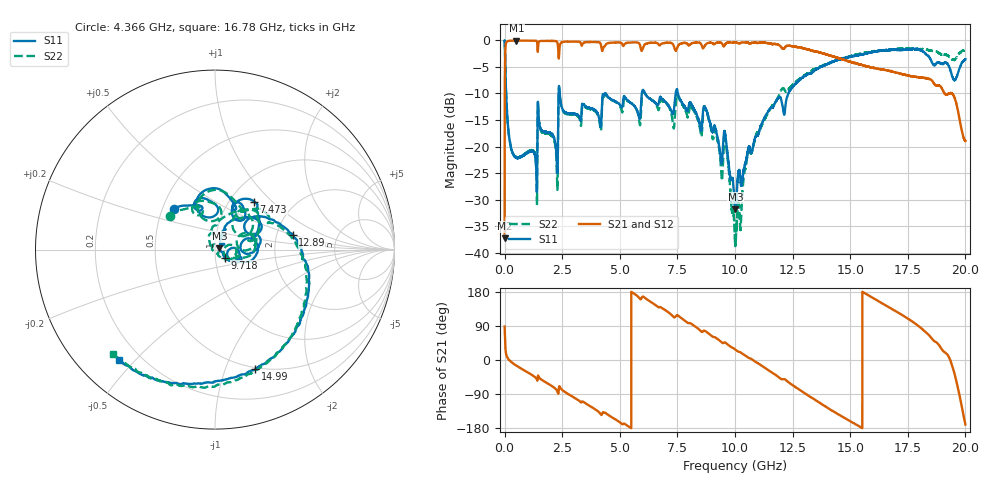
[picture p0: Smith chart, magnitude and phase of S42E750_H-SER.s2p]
!{S42E750}
!Johanson Technology Inc.
!www.johansontechnology.com
!Test Board Conditions:
!Substrate Type  RO4350B
!Substrate Thickness  50 mil
!Substrate Dk  3.66
!TL Type: GCPW
!TL Trace Width  60 mil
!TL Gap  10 mil
!Electrode orientation  Horizontal
!DUT TOPOLOGY	SERIES
!Mounting Pad LxW  14x55 mil
! Created Wed Nov 25 22:25:57 2020
# khz S ma R 50
! 2 Port Network Data from SP1.SP block
! freq  magS11  angS11  magS21  angS21  magS12  angS12  magS22  angS22
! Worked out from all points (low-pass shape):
!   20001 points, 300 kHz to 20 GHz, reference 50 ohm
!   highest |S21| = -0.04 dB at 511.3 MHz (marker M1); lowest = -37.3 dB at 300 kHz (marker M2)
!   |S21| within 3 dB of the highest: 21.74 MHz to 2.342 GHz (2.32 GHz wide, 196 % of centre); 2.36 GHz to 14.25 GHz (11.89 GHz wide, 143 % of centre)
!   lowest |S11| = -31.8 dB at 10.02 GHz (marker M3), VSWR 1.05, Z = 52.5 + j0.76 ohm
!   |S11| at or under -10 dB: 65.96 MHz to 2.345 GHz (2.279 GHz wide, 189 % of centre); 2.393 GHz to 4.351 GHz (1.958 GHz wide, 58.1 % of centre); 7.508 GHz to 12.31 GHz (4.806 GHz wide, 48.5 % of centre)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
!   |S22| runs from -38.7 to 0.0 dB; largest |S21 - S12| = 0.017
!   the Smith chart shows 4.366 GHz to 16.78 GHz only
!   S11 on the Smith chart (normalised r, x): 4.366 GHz: 0.58, +0.29; 7.473 GHz: 1.29, +0.78; 9.718 GHz: 1.11, -0.10; 12.89 GHz: 2.46, +0.50; 14.99 GHz: 0.49, -1.28; 16.78 GHz: 0.12, -0.45
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300  0.997 -0.9  0.0137 88.4  0.01378 89.2  0.9945 -0.9
110300  0.2001 -83.0  0.978 7.4  0.9787 7.3  0.2013 -82.9
511300  0.07853 -106.2  0.9957 -14.8  0.9946 -14.8  0.07943 -105.7
2125300  0.1239 -159.1  0.9869 -71.9  0.9868 -71.8  0.1192 -163.0
2431300  0.2653 -162.0  0.939 -74.6  0.9401 -74.7  0.2593 -158.2
3334300  0.2023 177.4  0.8996 -111.9  0.8997 -111.9  0.1782 -173.1
4366300  0.3194 135.2  0.894 -139.3  0.8933 -139.2  0.3135 143.8
6667300  0.2469 65.9  0.9288 139.5  0.9263 139.5  0.2222 51.1
7473300  0.3452 50.9  0.8306 118.2  0.8296 118.2  0.3069 45.5
8731300  0.2277 -9.8  0.9136 75.6  0.9136 75.5  0.2213 0.5
9718300  0.07068 -39.2  0.9607 39.3  0.9609 39.2  0.06552 -49.2
1.00003e7  0.02678 2.8  0.9618 28.1  0.9618 28.1  0.01249 -111.1
1.00213e7  0.02575 16.3  0.9609 27.1  0.9622 27.1  0.01204 -141.8
1.09413e7  0.1266 62.7  0.9461 -6.8  0.9462 -6.8  0.1328 92.6
1.28943e7  0.441 10.7  0.8493 -82.3  0.8474 -82.4  0.4493 5.2
1.33343e7  0.4917 -6.1  0.7973 -99.8  0.8011 -99.7  0.5208 -12.4
1.49933e7  0.7013 -71.2  0.6306 -161.2  0.6274 -161.5  0.7076 -70.6
1.66673e7  0.8099 -127.4  0.5199 139.9  0.5076 140.2  0.8124 -130.5
1.67773e7  0.8151 -131.0  0.5145 135.8  0.5005 136.2  0.8155 -134.4
1.78273e7  0.824 -174.2  0.4564 95.8  0.4598 96.5  0.8347 -169.2
1.89513e7  0.6012 148.7  0.362 30.6  0.3605 30.5  0.7353 157.4
2e7  0.6654 139.4  0.1125 -170.2  0.1126 -169.8  0.8061 127.6
